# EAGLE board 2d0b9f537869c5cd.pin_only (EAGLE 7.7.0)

Size 17.78 x 17.78 mm. Coordinates in mm from the lower left corner, seen from the top.
Outline: 0,0 0,17.78 17.78,17.78 17.78,0 0,0
Copper layers (1*16): Top 0.035mm / dielectric 1.5mm / Bottom 0.035mm
Design rules "SparkFun-2-layer-TIGHT": minimum track width 7mil, minimum drill 15mil, track to track 7mil, track to pad 7mil, pad to pad 7mil, via to via 7mil, smd to smd 7mil, copper to edge 7mil, drill to drill 7mil, minimum pad ring 7mil, minimum via ring 7mil, stop-mask expansion 4mil, vias tented up to drill 25mil, thermal gap 10mil

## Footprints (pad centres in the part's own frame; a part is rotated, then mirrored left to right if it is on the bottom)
0603 = smd 1.1 x 1: 1 -0.85,0; 2 0.85,0
FIDUCIAL-1X2 = smd 1 x 1: 1 0,0
STAND-OFF = hole 3.302: 0,0
1X03_NO_SILK = drill 1.016 pad 1.88: 1 0,0; 2 2.54,0; 3 5.08,0
1X04_NO_SILK = drill 1.016 pad 1.88: 1 0,0; 2 2.54,0; 3 5.08,0; 4 7.62,0
SMT-JUMPER_3_2-NC_TRACE_SILK = smd 0.635 x 1.27: 1 -1.016,0; 2 0,0; 3 1.016,0
SMT-JUMPER_2_NO_SILK = smd 0.635 x 1.27: 1 -0.406,0; 2 0.406,0
AXIAL-0.1 = drill 0.9 pad 1.88: P$1 -1.27,0; P$2 1.27,0
LGA10 = smd 0.7 x 0.4: 1 -1.1,1.2; 2 -1.1,0.6; 3 -1.1,0; 4 -1.1,-0.6; 5 -1.1,-1.2; 6 1.1,-1.2; 7 1.1,-0.6; 8 1.1,0; 9 1.1,0.6; 10 1.1,1.2 | smd 1.1 x 2.45: EP 0,0

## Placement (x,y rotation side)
C2  1.0uF  [0603]  8.89,13.34 180 top
FD1  FIDUCIAL1X2  [FIDUCIAL-1X2]  4.83,16.89 0 top
FD2  FIDUCIAL1X2  [FIDUCIAL-1X2]  15.24,3.81 0 top
FRAME1  FRAME-LETTER  [CREATIVE_COMMONS]  not placed on the board
H2  STAND-OFF  [STAND-OFF]  2.54,15.24 0 top
H4  STAND-OFF  [STAND-OFF]  15.24,15.24 0 top
J2  [1X03_NO_SILK]  6.35,1.27 180 top
J8  [1X04_NO_SILK]  16.51,1.27 180 top
JP1  [SMT-JUMPER_3_2-NC_TRACE_SILK]  2.54,10.16 90 bottom
JP2  [SMT-JUMPER_2_NO_SILK]  6.35,10.16 270 bottom
LOGO1  SFE_LOGO_FLAME.2_INCH  [SFE_LOGO_FLAME_.2]  10.92,11.05 0 bottom
LOGO4  OSHW-LOGOS  [OSHW-LOGO-S]  8.89,7.62 0 bottom
R1  100k  [0603]  10.79,6.35 180 top
R2  4.7k  [0603]  6.99,6.35 180 top
R6  100k  [0603]  5.21,10.16 270 top
R10  10k  [0603]  12.7,10.16 270 top
R12  10k  [AXIAL-0.1]  15.24,10.16 270 top
R13  4.7k  [0603]  2.54,11.43 180 top
R14  4.7k  [0603]  2.54,8.89 180 top
U2  CCS811  [LGA10]  8.89,10.16 90 top

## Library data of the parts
C2 = SparkFun-Capacitors; PROD_ID: CAP-00868
FD1 FD2 FRAME1 LOGO1 LOGO4 = SparkFun-Aesthetics
H2 H4 = SparkFun-Hardware
J2 J8 = SparkFun-Connectors
JP1 JP2 = SparkFun-Jumpers
R1 R6 = SparkFun-Resistors; PROD_ID: RES-07828
R2 R13 R14 = SparkFun-Resistors; PROD_ID: RES-07857
R10 = SparkFun-Resistors; PROD_ID: RES-00824
R12 = CCS811_Breakout_Temp; PROD_ID: N/A; SF_ID: SEN-00250
U2 = CCS811_Breakout_Temp; PROD_ID: IC-13607

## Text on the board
Bottom: v10
tPlace: CCS811 | Air Quality | NTC | !RST | !INT | !WAK | SCL | SDA | 3.3V | GND
bPlace: I2C PU | ADDR | !RST | !INT | !WAK | SCL | SDA | 3.3V | GND
Measures: All measurements in inches
tDocu: Nathan Seidle

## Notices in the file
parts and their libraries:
SparkFun-Aesthetics: Licensing: Creative Commons ShareAlike 4.0 International - https://creativecommons.org/licenses/by-sa/4.0
SparkFun-Aesthetics: Released under the Creative Commons Attribution Share-Alike 4.0 License
SparkFun-Aesthetics: https://creativecommons.org/licenses/by-sa/4.0
